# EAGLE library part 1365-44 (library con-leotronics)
DUAL ROW STRAIGHT HEADER 1364 SERIES. 1.27mm x 1.27mm. Without Fixing Post. SMT Source: http://www.leotronics.co.uk/Conexcon/Data%20Sheets/sec.%20A/1364ing.pdf
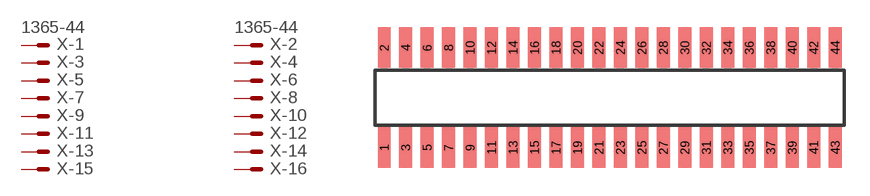
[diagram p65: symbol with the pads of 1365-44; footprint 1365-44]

Designator prefix X; gates -1=MVAL -2=MVAL -3=M -4=M -5=M -6=M -7=M -8=M -9=M -10=M -11=M -12=M -13=M -14=M -15=M -16=M -17=M -18=M -19=M -20=M -21=M -22=M -23=M -24=M -25=M -26=M -27=M -28=M -29=M -30=M -31=M -32=M -33=M -34=M -35=M -36=M -37=M -38=M -39=M -40=M -41=M -42=M -43=M -44=M

## 1365-44 (OC_FARNELL: unknown; OC_NEWARK: unknown)  [1365-44]
1  -1:S  pas
2  -2:S  pas
3  -3:S  pas
4  -4:S  pas
5  -5:S  pas
6  -6:S  pas
7  -7:S  pas
8  -8:S  pas
9  -9:S  pas
10  -10:S  pas
11  -11:S  pas
12  -12:S  pas
13  -13:S  pas
14  -14:S  pas
15  -15:S  pas
16  -16:S  pas
17  -17:S  pas
18  -18:S  pas
19  -19:S  pas
20  -20:S  pas
21  -21:S  pas
22  -22:S  pas
23  -23:S  pas
24  -24:S  pas
25  -25:S  pas
26  -26:S  pas
27  -27:S  pas
28  -28:S  pas
29  -29:S  pas
30  -30:S  pas
31  -31:S  pas
32  -32:S  pas
33  -33:S  pas
34  -34:S  pas
35  -35:S  pas
36  -36:S  pas
37  -37:S  pas
38  -38:S  pas
39  -39:S  pas
40  -40:S  pas
41  -41:S  pas
42  -42:S  pas
43  -43:S  pas
44  -44:S  pas

## Footprint 1365-44 (pad centres in mm)
DUAL ROW STRAIGHT HEADER 1364 SERIES. 1.27mm x 1.27mm. Without Fixing Post. SMT Source: http://www.leotronics.co.uk/Conexcon/Data%20Sheets/sec.%20A/1364ing.pdf
smd 0.76 x 2.4: 1 -13.335,-2.95; 2 -13.335,2.95; 3 -12.065,-2.95; 4 -12.065,2.95; 5 -10.795,-2.95; 6 -10.795,2.95; 7 -9.525,-2.95; 8 -9.525,2.95; 9 -8.255,-2.95; 10 -8.255,2.95; 11 -6.985,-2.95; 12 -6.985,2.95; 13 -5.715,-2.95; 14 -5.715,2.95; 15 -4.445,-2.95; 16 -4.445,2.95; 17 -3.175,-2.95; 18 -3.175,2.95; 19 -1.905,-2.95; 20 -1.905,2.95; 21 -0.635,-2.95; 22 -0.635,2.95; 23 0.635,-2.95; 24 0.635,2.95; 25 1.905,-2.95; 26 1.905,2.95; 27 3.175,-2.95; 28 3.175,2.95; 29 4.445,-2.95; 30 4.445,2.95; 31 5.715,-2.95; 32 5.715,2.95; 33 6.985,-2.95; 34 6.985,2.95; 35 8.255,-2.95; 36 8.255,2.95; 37 9.525,-2.95; 38 9.525,2.95; 39 10.795,-2.95; 40 10.795,2.95; 41 12.065,-2.95; 42 12.065,2.95; 43 13.335,-2.95; 44 13.335,2.95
